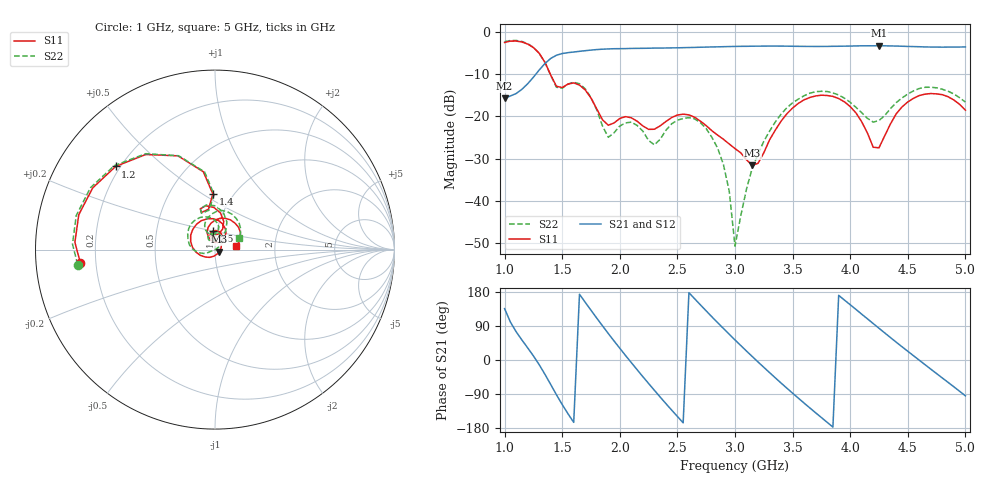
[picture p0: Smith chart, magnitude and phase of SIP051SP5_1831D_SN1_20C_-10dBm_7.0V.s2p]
# GHz  S  dB  R  50
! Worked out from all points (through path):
!   81 points, 1 GHz to 5 GHz, reference 50 ohm
!   highest |S21| = -3.23 dB at 4.25 GHz (marker M1); lowest = -15.7 dB at 1 GHz (marker M2)
!   lowest |S11| = -31.6 dB at 3.15 GHz (marker M3), VSWR 1.05, Z = 52.4 - j1.28 ohm
!   |S11| at or under -10 dB: 1.397 GHz to end of sweep
!   |S22| runs from -50.8 to -2.0 dB; largest |S21 - S12| = 0.0036
!   S11 on the Smith chart (normalised r, x): 1 GHz: 0.14, -0.05; 1.2 GHz: 0.18, +0.35; 1.4 GHz: 0.81, +0.55; 2.5 GHz: 0.96, +0.20; 5 GHz: 1.26, +0.05
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1  -2.46 -174.3  -15.70 135.5  -15.71 135.4  -2.27 -173.8
1.2  -2.83 140.0  -12.27 32.2  -12.28 32.2  -2.73 140.1
1.4  -10.17 92.2  -6.25 -64.5  -6.25 -64.5  -10.26 91.0
1.5  -13.15 110.1  -5.08 -117.5  -5.08 -117.5  -13.32 110.5
1.7  -13.73 81.2  -4.41 152.2  -4.42 152.2  -13.45 77.4
1.85  -20.81 75.7  -4.05 90.2  -4.06 90.2  -22.29 62.8
2.05  -20.06 99.9  -3.92 11.7  -3.92 11.8  -21.55 101.3
2.2  -22.27 91.1  -3.85 -44.0  -3.84 -43.7  -23.50 84.7
2.35  -22.25 108.6  -3.78 -97.6  -3.78 -97.5  -25.46 120.4
2.5  -19.68 96.9  -3.73 -148.9  -3.73 -149.0  -20.91 110.7
2.65  -20.22 70.5  -3.63 161.5  -3.63 161.4  -20.59 77.8
2.85  -24.46 48.3  -3.50 98.3  -3.50 98.4  -27.59 40.7
2.95  -26.56 39.4  -3.43 68.0  -3.43 67.9  -37.75 32.8
3  -27.64 32.7  -3.40 52.9  -3.40 52.9  -50.80 19.6
3.15  -31.60 -27.6  -3.34 9.2  -3.35 9.1  -32.27 -157.7
3.45  -19.39 -172.7  -3.33 -74.3  -3.33 -74.3  -17.95 178.0
3.7  -15.15 126.1  -3.40 -139.4  -3.40 -139.4  -14.14 132.1
3.95  -16.55 73.2  -3.33 158.2  -3.34 158.2  -15.68 90.8
4.25  -27.46 96.5  -3.23 83.8  -3.24 83.6  -20.98 107.3
4.35  -21.77 117.7  -3.29 59.1  -3.29 59.2  -18.16 115.9
4.65  -14.72 71.6  -3.52 -12.5  -3.51 -12.4  -13.10 79.7
5  -18.53 9.8  -3.52 -94.6  -3.53 -94.4  -16.62 25.5
